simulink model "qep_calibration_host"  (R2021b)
settings: Solver=FixedStepDiscrete  StartTime=0.0  StopTime=Inf  RelTol=1e-3
undefined symbols (not defined in the file or in its folder): motor, Serial
libraries: mcbhostblockslib x3, simulink x1

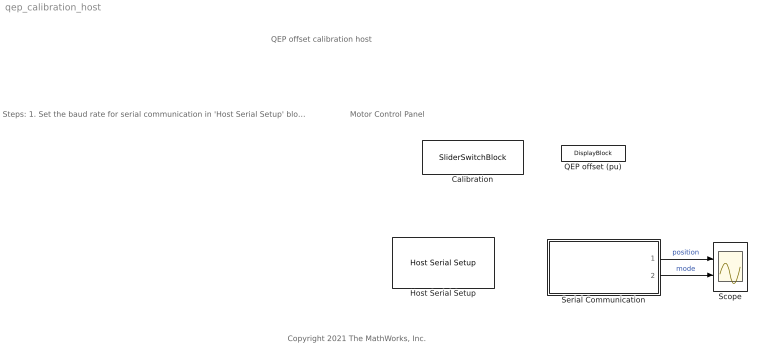
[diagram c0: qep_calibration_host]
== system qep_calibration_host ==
  note: QEP offset calibration host
  note: Motor Control Panel
  note: Steps: 1. Set the baud rate for serial communication in 'Host Serial Setup' block. 2. Select the serial port in ' Serial 1 ' tab of ' Host Serial Setup ' block. 3. Use ' Calibration Start / Stop ' switch to control the motor. 4. Observe the position signal on the scope and ensure that the signal has a positive slope. If not, stop the calibration, disconnect the power supply and interchange two of the motor phases. 5. The calculated offset will be displayed on the "QEP offset (pu)" block
  note: Copyright 2021 The MathWorks, Inc.
  Calibration : SliderSwitchBlock  LabelPosition=Hide
  Host Serial Setup : mcbhostblockslib/Host Serial Setup  Priority=-99  comPortSer1='Please_select_a_port'  baudRateA=4000000  charLenA=8  stopBitA=1  parityA=none  timeoutA=2.0  ByteOrderA=LittleEndian  comPortSer2='Please_select_a_port'  baudRateB=115200  charLenB=8  stopBitB=1  parityB=none  timeoutB=1.0  ByteOrderB=LittleEndian  comPortSer3='Please_select_a_port'  baudRateC=115200  charLenC=8  stopBitC=1  parityC=none  timeoutC=1.0  ByteOrderC=LittleEndian  comPortSer4='Please_select_a_port'  baudRateD=115200  charLenD=8  stopBitD=1  parityD=none  timeoutD=1.0  ByteOrderD=LittleEndian
  QEP offset (pu) : DisplayBlock  LabelPosition=Hide  Format=short  Transparency=1
  Scope : Scope  NumInputPorts=2
  Serial Communication : Subsystem
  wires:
  Serial Communication/1(position) -> Scope/1  "position"
  Serial Communication/2(mode) -> Scope/2  "mode"

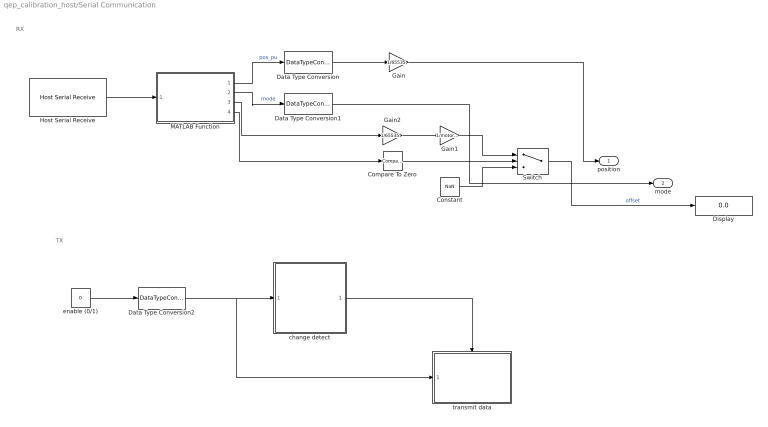
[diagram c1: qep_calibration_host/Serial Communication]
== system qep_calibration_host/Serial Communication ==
  note: TX
  note: RX
  Compare To Zero : simulink/Logic and Bit Operations/Compare To Zero  relop=>  OutDataTypeStr=boolean
  Constant : Constant  Value=NaN  OutDataTypeStr=single
  Data Type Conversion : DataTypeConversion  OutDataTypeStr=single
  Data Type Conversion1 : DataTypeConversion  OutDataTypeStr=single
  Data Type Conversion2 : DataTypeConversion  OutDataTypeStr=single
  Display : Display
  Gain : Gain  Gain=1/65535  OutDataTypeStr=single
  Gain1 : Gain  Gain=1/motor.polepairs  OutDataTypeStr=single
  Gain2 : Gain  Gain=1/65535  OutDataTypeStr=single
  Host Serial Receive : mcbhostblockslib/Host Serial Receive  serialCon=Serial 1  dataHead='ss'  dataTail='ee'  dataType=uint16  dataDim=[200 2]  initValue=2000  errOption=Output custom value  errValue=4000  sampleTime=200 * 50e-6  outputStatus=off  blockingMode=on
  MATLAB Function : MATLAB Function  TreatAsAtomicUnit=on
  Switch : Switch  Criteria=u2 > Threshold
  change detect : Subsystem
  enable (0/1) : Constant  Value=0  OutDataTypeStr=boolean  SampleTime=-1
  transmit data : Subsystem  TreatAsAtomicUnit=on
  position : Outport
  mode : Outport  Port=2
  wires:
  Gain/1 -> position/1
  Data Type Conversion1/1 -> mode/1
  Switch/1 -> Display/1  "offset"
  Data Type Conversion/1 -> Gain/1
  Gain1/1 -> Switch/1
  MATLAB Function/2(Output2) -> Data Type Conversion1/1  "mode"
  Compare To Zero/1 -> Switch/2
  MATLAB Function/3(Output3) -> Gain2/1
  MATLAB Function/4(Output4) -> Compare To Zero/1
  Gain2/1 -> Gain1/1
  Host Serial Receive/1 -> MATLAB Function/1(Input)
  Constant/1 -> Switch/3
  MATLAB Function/1(Output1) -> Data Type Conversion/1  "pos_pu"
  Data Type Conversion2/1 -> transmit data/1(enable), change detect/1(enable)
  change detect/1(isChange) -> transmit data/Enable
  enable (0/1)/1 -> Data Type Conversion2/1

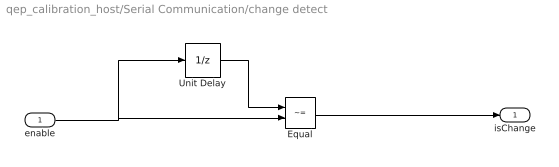
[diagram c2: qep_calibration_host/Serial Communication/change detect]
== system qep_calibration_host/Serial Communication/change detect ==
  enable : Inport
  Equal : RelationalOperator  Operator=~=  OutDataTypeStr=boolean  RndMeth=Simplest
  Unit Delay : UnitDelay  SampleTime=-1  HasFrameUpgradeWarning=on
  isChange : Outport
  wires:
  Unit Delay/1 -> Equal/1
  enable/1 -> Equal/2, Unit Delay/1
  Equal/1 -> isChange/1

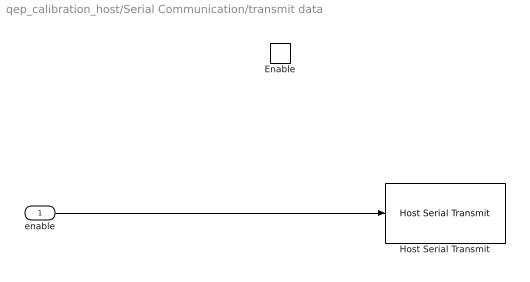
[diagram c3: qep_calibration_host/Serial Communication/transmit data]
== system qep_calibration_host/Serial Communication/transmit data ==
  enable : Inport
  Enable : EnablePort
  Host Serial Transmit : mcbhostblockslib/Host Serial Transmit  serialCon=Serial 1  header=''  tail=''  enableBlockingMode=off
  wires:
  enable/1 -> Host Serial Transmit/1

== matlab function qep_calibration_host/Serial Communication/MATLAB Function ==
function [Output1, Output2, Output3, Output4]  = unBuf(Input)

Output1 = Input(:, 1);
Output2 = Input(:, 2);
Output3 = Output1(1);
Output4 = Output2(1);

end
